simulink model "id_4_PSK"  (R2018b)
settings: Solver=VariableStepAuto  StartTime=0.0  StopTime=inf  RelTol=1e-3
libraries: commdigbbndpm3 x2, commfilt2 x2, commchan3 x1, commrandsrc3 x1, commsink2 x1, commutil2 x1

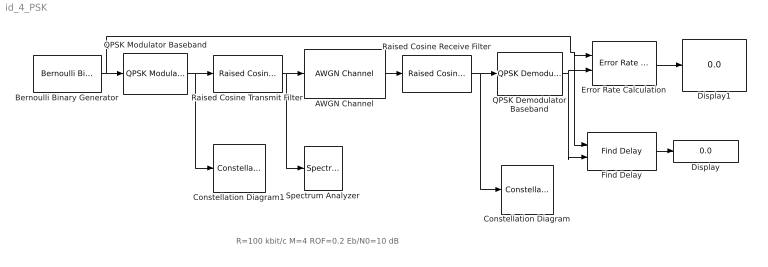
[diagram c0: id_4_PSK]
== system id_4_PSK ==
  note: R=100 kbit/c M=4 ROF=0.2 Eb/N0=10 dB
  AWGN Channel : commchan3/AWGN Channel  InputProcessing=Columns as channels (frame based)  seed=67  noiseMode="Signal to noise ratio  (Eb/No)"  EbNodB=10  EsNodB=10  SNRdB=10  bitsPerSym=2  Ps=1/8  Tsym=1/50e3  variance=1
  Bernoulli Binary Generator : commrandsrc3/Bernoulli Binary Generator  ProbabilityOfZero=0.5  SeedSource=Auto  Seed=0  SampleTime=1/100e3  SamplesPerFrame=200  OutputDataType=double  SimulateUsing=Interpreted execution
  Constellation Diagram : ConstellationDiagram
  Constellation Diagram1 : ConstellationDiagram
  Display : Display
  Display1 : Display
  Error Rate Calculation : commsink2/Error Rate Calculation  N=20  st_delay=0  cp_mode=Entire frame  subframe=[]  PMode=Port  WsName=ErrorVec  RsMode2=off  stop=off  numErr=100  maxBits=1e6
  Find Delay : commutil2/Find Delay  corrLength=200  chgSigOP=off  stopUpdate=on  numConstDelay=10
  QPSK Demodulator Baseband : commdigbbndpm3/QPSK Demodulator Baseband  OutType=Bit  DecType=Hard decision  VarSource=Dialog  Variance=1  Dec=Gray  Ph=pi/4  outDtype1=Inherit via internal rule  outDtype2=Inherit via internal rule  derotateFactorWordLen=16  derotateFactorDataTypeStr=Inherit: Same word length as input  derotateFactorLastDataTypeStr=Inherit: Same word length as input
  QPSK Modulator Baseband : commdigbbndpm3/QPSK Modulator Baseband  InType=Bit  Enc=Gray  Ph=pi/4  outDtype=double  outWordLen=16  outUDDataType=sfix(16)  outFracLenMode=Best precision  outFracLen=15  outDataTypeStr=double  outLastDataTypeStr=double
  Raised Cosine Receive Filter : commfilt2/Raised Cosine Receive Filter  filtType=Square root  R=0.2  filtSpan=10  N=8  downFactor=8  downOffset=0  filterGain=1  InputProcessing=Columns as channels (frame based)  RateOptions=Enforce single-rate processing  framing=Mute  checkCoeff=off  variableName=rcRxFilt  currentFiltSpan=10  D=5  inputOffset=0  sampMode=Mute  saveAsFlag=0  rateMode=Downsampling  checkGain=Normalized  launchFVT=on  roundingMode=Floor  overflowMode=off  coeffDataTypeStr=Inherit: Same word length as input  coeffMin=[]  coeffMax=[]  coeffLastDataTypeStr=Inherit: Same word length as input  accumDataTypeStr=Inherit: Same as product output  accumLastDataTypeStr=Inherit: Same as product output  outputDataTypeStr=Inherit: Same as accumulator  outputMin=[]  outputMax=[]  outputLastDataTypeStr=Inherit: Same as accumulator
  Raised Cosine Transmit Filter : commfilt2/Raised Cosine Transmit Filter  filtType=Square root  R=0.2  filtSpan=10  N=8  filterGain=1  InputProcessing=Columns as channels (frame based)  RateOptions=Enforce single-rate processing  framing=Mute  checkCoeff=off  variableName=rcTxFilt  checkGain=Normalized  sampMode=Mute  saveAsFlag=0  currentFiltSpan=10  D=5  launchFVT=on  roundingMode=Floor  overflowMode=off  coeffDataTypeStr=Inherit: Same word length as input  coeffMin=[]  coeffMax=[]  coeffLastDataTypeStr=Inherit: Same word length as input  outputDataTypeStr=Inherit: Same as accumulator  outputMin=[]  outputMax=[]  outputLastDataTypeStr=Inherit: Same as accumulator
  Spectrum Analyzer : SpectrumAnalyzer
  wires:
  Bernoulli Binary Generator/1 -> Find Delay/1, Error Rate Calculation/1, QPSK Modulator Baseband/1
  QPSK Modulator Baseband/1 -> Constellation Diagram1/1, Raised Cosine Transmit Filter/1
  AWGN Channel/1 -> Raised Cosine Receive Filter/1
  QPSK Demodulator Baseband/1 -> Find Delay/2, Error Rate Calculation/2
  Error Rate Calculation/1 -> Display1/1
  Find Delay/1 -> Display/1
  Raised Cosine Receive Filter/1 -> Constellation Diagram/1, QPSK Demodulator Baseband/1
  Raised Cosine Transmit Filter/1 -> Spectrum Analyzer/1, AWGN Channel/1
